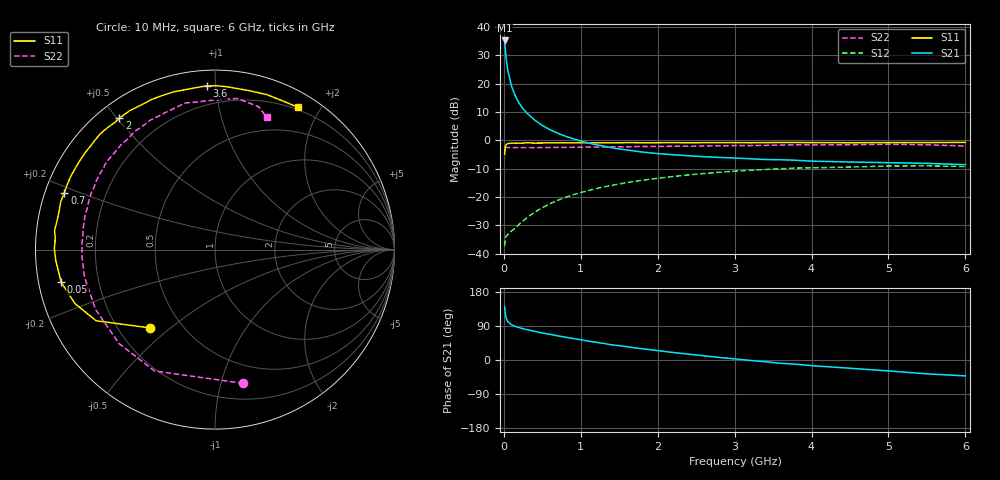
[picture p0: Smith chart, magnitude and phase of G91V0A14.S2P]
! SIEMENS Small Signal Semiconductors
! BFG235
! Si NPN RF Bipolar Junction Transistor in SOT223
! VCE = 1 V  IC = 140 mA
! Common Emitter S-Parameters:  July  1994
# GHz  S  MA  R  50
!  f  S11  S21  S12  S22
! GHz  MAG  ANG  MAG  ANG  MAG  ANG  MAG  ANG
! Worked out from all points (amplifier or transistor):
!   40 points, 10 MHz to 6 GHz, reference 50 ohm
!   highest |S21| = 35.2 dB at 10 MHz (marker M1)
!   |S21| within 3 dB of that: start of sweep to 18.68 MHz
!   unconditionally stable (mu >= 1): 391 MHz to 2.046 GHz
!   at 200 MHz: K = 0.83, MSG = 21.3 dB, |S12| = -29.6 dB
!   at 1.5 GHz: K = 1.02, MAG = 5.3 dB, |S12| = -15.4 dB
!   at 6 GHz: K = 0.95, MSG = 0.3 dB, |S12| = -9.3 dB
!   S11 on the Smith chart (normalised r, x): 10 MHz: 0.33, -0.43; 50 MHz: 0.07, -0.10; 700 MHz: 0.06, +0.18; 2 GHz: 0.06, +0.51; 3.6 GHz: 0.09, +0.95; 6 GHz: 0.17, +1.73
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0.01  0.5662 -129.6  57.45 140.1  0.0136 49.4  0.7618 -78.0
0.02  0.772 -149.1  38.58 120.3  0.0184 35.1  0.7557 -116.5
0.03  0.8361 -158.9  27.88 110.5  0.0202 30.1  0.7482 -135.6
0.05  0.8758 -168.0  17.51 101.4  0.0218 27.2  0.7441 -153.3
0.1  0.8893 -176.1  8.973 93.1  0.0251 34.0  0.7433 -168.1
0.15  0.8952 179.6  5.989 88.4  0.0284 41.7  0.7403 -174.3
0.2  0.8923 177.5  4.473 85.4  0.0333 46.8  0.7431 -177.8
0.25  0.8945 175.0  3.608 82.5  0.038 51.2  0.7407 179.5
0.3  0.9002 173.2  3.016 80.3  0.0431 54.0  0.7419 177.2
0.4  0.8937 169.0  2.277 75.6  0.0539 57.4  0.7401 173.7
0.5  0.8956 165.4  1.826 71.4  0.0649 58.4  0.7438 170.7
0.7  0.8973 159.3  1.333 63.8  0.0876 58.2  0.7488 165.0
0.9  0.9011 153.8  1.064 56.7  0.1093 55.8  0.7516 160.1
1.1  0.9012 147.3  0.893 49.6  0.1303 52.9  0.7582 155.2
1.4  0.9019 140.2  0.739 40.2  0.1599 47.6  0.7658 148.5
2  0.9058 126.1  0.584 24.8  0.2135 36.0  0.7776 136.0
2.2  0.9083 121.6  0.556 19.8  0.2297 32.2  0.7845 131.9
3.2  0.9062 100.7  0.472 -1.1  0.2955 12.8  0.8071 113.1
3.6  0.914 92.8  0.454 -8.6  0.3148 4.5  0.8216 105.1
4.5  0.9058 78.0  0.414 -21.8  0.3378 -10.9  0.8341 89.9
5.5  0.9104 65.2  0.392 -36.6  0.3543 -28.1  0.8323 73.0
6  0.9182 59.6  0.371 -42.0  0.3441 -34.5  0.7919 68.7
